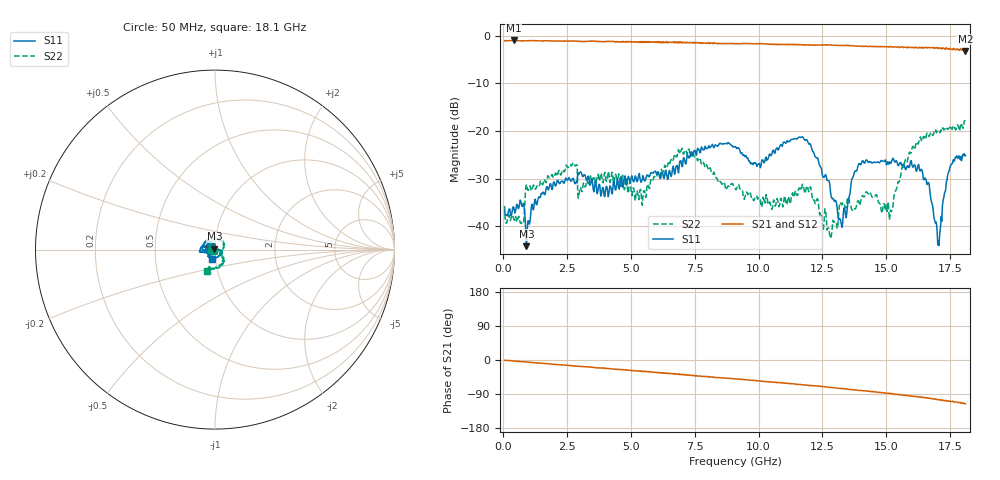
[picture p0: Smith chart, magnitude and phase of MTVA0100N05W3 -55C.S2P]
! Network Analyzer HP8720D.06.14 Serial No. US36140669
! 17 Jan 2005  08:56:33
! Frequency  S11  S21  S12  S22
# HZ  S  DB R 50
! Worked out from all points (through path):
!   801 points, 50 MHz to 18.1 GHz, reference 50 ohm
!   highest |S21| = -1.02 dB at 411 MHz (marker M1); lowest = -3.2 dB at 18.1 GHz (marker M2)
!   group delay of S21, straight-line fit = 16.8 ps
!   lowest |S11| = -44.1 dB at 907.4 MHz (marker M3), VSWR 1.01, Z = 49.7 + j0.516 ohm
!   |S11| at or under -10 dB: start of sweep to end of sweep
!   |S22| runs from -42.5 to -17.8 dB; largest |S21 - S12| = 0.028
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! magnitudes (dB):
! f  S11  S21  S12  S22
! 50 MHz  -36.7  -1.1  -1.1  -35.7
! 411 MHz  -36.1  -1.0  -1.0  -38.4
! 726.9 MHz  -35.7  -1.1  -1.1  -39.2
! 907.4 MHz  -44.1  -1.1  -1.1  -31.2
! 1.765 GHz  -32.3  -1.1  -1.1  -29.5
! 2.69 GHz  -30.2  -1.1  -1.1  -27.1
! 3.073 GHz  -29.0  -1.2  -1.2  -32.7
! 3.886 GHz  -31.9  -1.3  -1.3  -30.7
! 5.51 GHz  -30.3  -1.4  -1.4  -32.5
! 6.074 GHz  -28.7  -1.4  -1.4  -29.1
! 7.202 GHz  -25.0  -1.4  -1.5  -24.8
! 9.075 GHz  -23.3  -1.7  -1.7  -31.9
! 10 GHz  -26.9  -1.7  -1.7  -33.9
! 12.1 GHz  -23.9  -1.9  -2.0  -33.7
! 12.78 GHz  -30.8  -2.0  -1.9  -41.5
! 13.2 GHz  -38.5  -2.1  -2.1  -34.9
! 13.99 GHz  -27.1  -2.2  -2.3  -34.8
! 15.1 GHz  -26.9  -2.4  -2.3  -36.8
! 16.34 GHz  -28.3  -2.5  -2.5  -21.2
! 17.04 GHz  -43.1  -2.6  -2.7  -19.8
! 17.49 GHz  -27.6  -2.7  -2.6  -18.9
! 18.1 GHz  -25.2  -3.2  -3.1  -17.9
